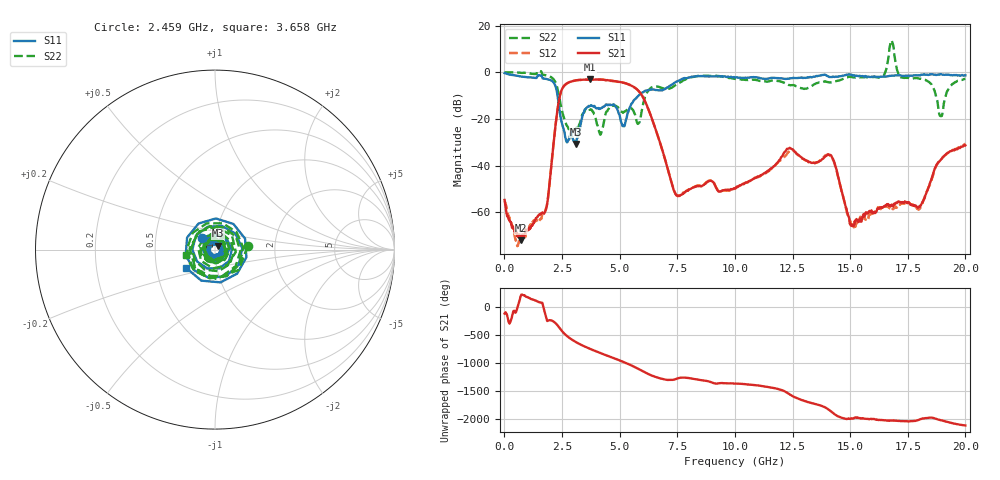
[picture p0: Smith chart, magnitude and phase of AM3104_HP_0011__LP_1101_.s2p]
!Created with skrf (http://scikit-rf.org).
# Hz S RI R 50.0
!freq ReS11 ImS11 ReS21 ImS21 ReS12 ImS12 ReS22 ImS22
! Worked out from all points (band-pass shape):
!   1601 points, 10 MHz to 20 GHz, reference 50 ohm
!   highest |S21| = -3.09 dB at 3.708 GHz (marker M1); lowest = -71.9 dB at 722.1 MHz (marker M2)
!   |S21| within 3 dB of the highest: 2.571 GHz to 5.574 GHz (3.003 GHz wide, 73.8 % of centre)
!   lowest |S11| = -30.7 dB at 3.121 GHz (marker M3), VSWR 1.06, Z = 51.8 + j2.33 ohm
!   |S11| at or under -10 dB: 2.305 GHz to 5.815 GHz (3.51 GHz wide, 86.4 % of centre)
!   |S22| runs from -26.7 to 13.6 dB; largest |S21 - S12| = 0.07
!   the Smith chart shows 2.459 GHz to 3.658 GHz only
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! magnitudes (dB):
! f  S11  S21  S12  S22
! 10 MHz  -0.4  -54.7  -55.1  0.0
! 722.1 MHz  -1.8  -71.9  -72.8  -0.3
! 1.784 GHz  -2.8  -59.4  -59.1  -1.3
! 2.421 GHz  -18.3  -9.5  -9.6  -12.9
! 3.121 GHz  -30.7  -3.4  -3.4  -23.9
! 3.346 GHz  -20.5  -3.2  -3.3  -19.5
! 3.708 GHz  -14.5  -3.1  -3.2  -16.1
! 4.158 GHz  -15.6  -3.1  -3.2  -26.7
! 5.157 GHz  -22.9  -4.4  -4.5  -17.3
! 5.732 GHz  -10.9  -7.1  -7.2  -20.9
! 6.682 GHz  -7.7  -28.0  -28.1  -6.2
! 7.506 GHz  -3.9  -52.8  -53.0  -5.0
! 10.01 GHz  -2.3  -49.8  -49.9  -2.9
! 12.33 GHz  -2.8  -32.7  -34.2  -5.5
! 13.34 GHz  -2.2  -38.9  -38.8  -5.8
! 14.22 GHz  -2.1  -36.5  -36.8  -4.3
! 15.08 GHz  -1.1  -65.3  -65.5  -2.1
! 16.39 GHz  -1.9  -58.1  -58.3  -2.0
! 16.68 GHz  -1.6  -57.1  -58.1  7.3
! 18.03 GHz  -1.4  -57.3  -58.4  -2.8
! 18.93 GHz  -0.8  -37.6  -37.4  -18.8
! 20 GHz  -1.3  -31.3  -30.7  -2.8
